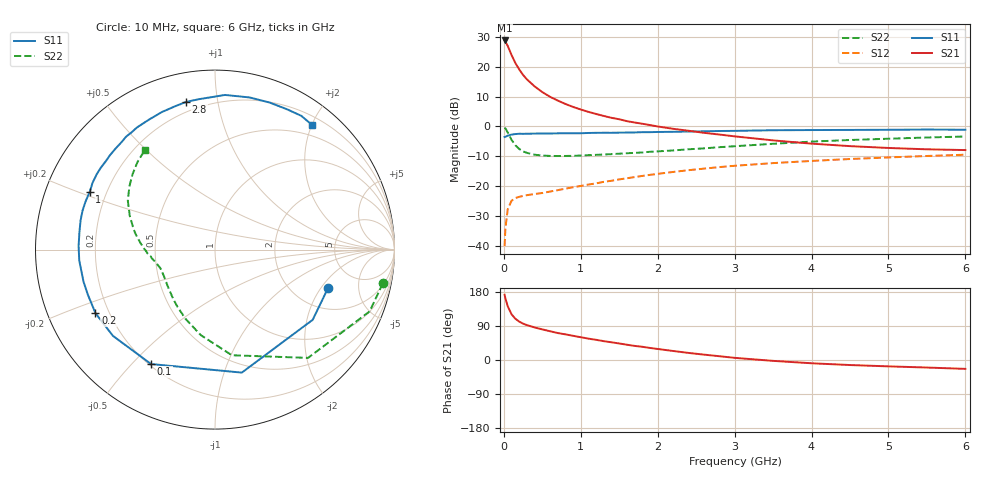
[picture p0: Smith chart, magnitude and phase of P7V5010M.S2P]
! SIEMENS Small Signal Semiconductors
! BFP196
! Si NPN RF Bipolar Junction Transistor in SOT143
! VCE = 0.5 V  IC = 10 mA
! Common Emitter S-Parameters:  May  1996
# GHz  S  MA  R  50
!  f  S11  S21  S12  S22
! GHz  MAG  ANG  MAG  ANG  MAG  ANG  MAG  ANG
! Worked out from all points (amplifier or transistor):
!   36 points, 10 MHz to 6 GHz, reference 50 ohm
!   highest |S21| = 28.8 dB at 10 MHz (marker M1)
!   |S21| within 3 dB of that: start of sweep to 69.65 MHz
!   unconditionally stable (mu >= 1): 828.5 MHz to end of sweep
!   at 250 MHz: K = 0.42, MSG = 20.3 dB, |S12| = -23.3 dB
!   at 1.4 GHz: K = 1.19, MAG = 7.9 dB, |S12| = -18.2 dB
!   at 6 GHz: K = 1.05, MAG = -0.6 dB, |S12| = -9.5 dB
!   S11 on the Smith chart (normalised r, x): 10 MHz: 3.06, -2.34; 100 MHz: 0.21, -0.57; 200 MHz: 0.15, -0.24; 1 GHz: 0.14, +0.22; 2.8 GHz: 0.15, +0.81; 6 GHz: 0.33, +2.01
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0.01  0.6654 -18.7  27.48 172.1  0.0099 82.0  0.9539 -11.4
0.02  0.6703 -35.7  26.3 162.7  0.0193 73.8  0.9277 -21.8
0.05  0.7014 -77.7  22.35 142.1  0.0408 55.6  0.7957 -49.3
0.1  0.7305 -119.2  15.71 120.7  0.057 38.1  0.5962 -80.9
0.15  0.7446 -139.8  11.49 108.8  0.0633 31.2  0.4827 -99.5
0.2  0.7542 -152.0  9.001 101.3  0.0663 28.0  0.4194 -113.0
0.25  0.7516 -160.5  7.279 96.0  0.0686 26.6  0.3817 -123.1
0.3  0.7541 -166.2  6.135 92.1  0.0707 26.3  0.3611 -130.0
0.4  0.7588 -175.5  4.68 85.9  0.074 27.2  0.3361 -140.5
0.5  0.7602 178.4  3.755 80.8  0.0768 28.7  0.3254 -147.6
0.6  0.7616 172.6  3.137 75.9  0.0812 30.5  0.3208 -152.4
0.7  0.7664 167.7  2.712 71.2  0.0857 32.0  0.3199 -155.9
0.8  0.7692 163.6  2.379 67.7  0.0909 33.3  0.3205 -158.7
1  0.7686 155.1  1.919 60.1  0.1009 35.8  0.3256 -163.2
1.1  0.7771 151.4  1.752 56.4  0.1064 36.6  0.3306 -165.0
1.6  0.7897 134.7  1.225 40.3  0.1356 37.7  0.3558 -172.4
2.2  0.8123 116.9  0.913 23.8  0.173 34.6  0.3962 179.0
2.8  0.8384 101.1  0.732 10.0  0.2084 29.2  0.4491 169.2
3.5  0.8634 86.3  0.584 -2.3  0.2433 21.3  0.5119 158.2
4.5  0.8739 69.7  0.468 -13.3  0.2848 10.3  0.5927 143.6
5.5  0.8869 57.2  0.414 -19.9  0.3203 -0.2  0.6527 131.3
6  0.8803 51.9  0.402 -23.4  0.3362 -6.0  0.6784 125.2
